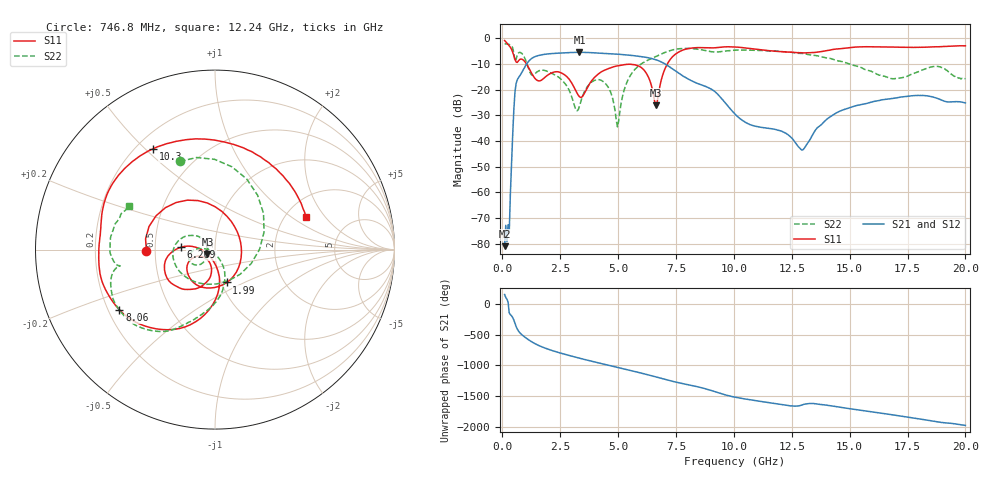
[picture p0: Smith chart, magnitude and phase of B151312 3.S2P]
!  2-Port S-parameters saved by WinCal
! VAR MeasName=S-Parameters (CALIBRATED_DATA) read from VNA (N5244A)
! VAR MeasDate=12/8/2015 5:44:01 PM
! VAR NAME=B151312 3
! VAR FILENAME=B151312 3.S2P
! VAR DATE=12/8/2015 5:44:01 PM
! VAR PHYS_PORTS=1,2
# Hz S DB R 50
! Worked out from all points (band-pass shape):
!   401 points, 100 MHz to 20 GHz, reference 50 ohm
!   highest |S21| = -5.52 dB at 3.334 GHz (marker M1); lowest = -80.9 dB at 100 MHz (marker M2)
!   |S21| within 3 dB of the highest: 1.189 GHz to 6.67 GHz (5.481 GHz wide, 139 % of centre)
!   lowest |S11| = -26.2 dB at 6.617 GHz (marker M3), VSWR 1.10, Z = 45.9 - j2.3 ohm
!   |S11| at or under -10 dB: 1.044 GHz to 7.131 GHz (6.088 GHz wide, 149 % of centre)
!   |S22| runs from -34.5 to -2.2 dB; largest |S21 - S12| = 0.0015
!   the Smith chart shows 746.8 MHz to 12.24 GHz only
!   S11 on the Smith chart (normalised r, x): 746.8 MHz: 0.45, -0.01; 1.99 GHz: 1.06, -0.40; 6.269 GHz: 0.68, +0.02; 8.06 GHz: 0.25, -0.27; 10.3 GHz: 0.27, +0.53; 12.24 GHz: 2.58, +1.30
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1e8  -0.91 -41.8  -80.92 148.2  -75.89 140.3  -2.19 169.3
2.4925e8  -2.41 -93.1  -72.57 26.4  -73.31 12.8  -2.36 152.1
5.4775e8  -8.24 -166.7  -20.95 41.7  -20.95 41.7  -9.08 114.8
7.4675e8  -8.35 -179.1  -14.77 -106.2  -14.77 -106.2  -5.53 111.6
1.34375e9  -14.84 59.7  -7.49 85.5  -7.49 85.5  -14.35 -87.2
1.9905e9  -14.21 -70.3  -6.12 -19.2  -6.12 -19.2  -13.09 172.3
2.63725e9  -13.97 -139.9  -5.74 -93.9  -5.74 -93.9  -16.92 146.7
3.33375e9  -22.79 -140.7  -5.52 -163.6  -5.52 -163.6  -26.39 -147.5
3.43325e9  -22.93 -122.9  -5.53 -173.1  -5.52 -173.1  -23.48 -136.1
4.279e9  -13.11 -110.9  -5.89 109.3  -5.88 109.2  -16.43 -164.9
4.9755e9  -10.79 -131.6  -6.24 47.8  -6.24 47.8  -34.55 -130.6
5.473e9  -10.15 -147.9  -6.63 3.3  -6.63 3.2  -15.48 -70.9
6.269e9  -14.43 176.0  -7.57 -70.7  -7.58 -70.8  -8.66 -101.6
6.61725e9  -26.20 -149.3  -8.36 -105.6  -8.36 -105.7  -7.27 -110.2
6.7665e9  -20.51 -85.6  -8.85 -121.0  -8.86 -121.0  -6.62 -113.8
8.06e9  -4.02 -147.8  -16.06 123.6  -16.06 123.4  -3.99 -153.3
1.005e10  -3.44 133.2  -29.52 -75.5  -29.59 -75.7  -4.68 -177.6
1.029875e10  -3.62 121.6  -31.52 -93.0  -31.57 -93.0  -4.66 178.9
1.2239e10  -5.39 19.5  -36.95 153.7  -37.02 154.0  -5.41 153.2
1.338325e10  -5.67 -31.3  -37.94 -177.6  -37.82 -177.0  -6.65 138.4
1.67165e10  -3.45 -114.0  -23.62 6.0  -23.45 5.7  -15.50 138.1
2e10  -2.99 -147.5  -25.22 -173.8  -25.23 -175.0  -15.79 137.4
